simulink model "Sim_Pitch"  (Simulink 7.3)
settings: Solver=ode45  StartTime=0.0  StopTime=50  RelTol=1e-3
StartFcn:
  | [Avp, Bvp, Cvp, Dvp]= vehi_pdes;
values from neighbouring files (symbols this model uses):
  d2r = pi/180    (= 0.0174532925199)    [run.m]
  r2d = 180/pi    (= 57.2957795131)    [Pl.m]    (also in run.m)
undefined symbols (not defined in the file or in its folder): Avp, Bvp, Cvp, Dvp

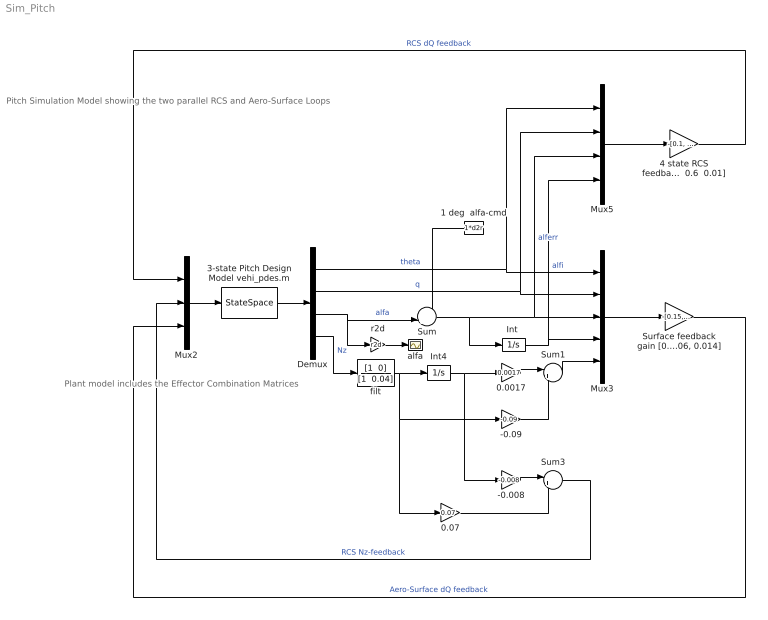
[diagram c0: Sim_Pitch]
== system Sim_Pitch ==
  note: Pitch Simulation Model showing the two parallel RCS and Aero-Surface Loops
  note: Plant model includes the Effector Combination Matrices
  -0.008 : Gain  Gain=-0.008  ParameterDataType=sfix(16)  ParameterScaling=2^0  OutDataType=sfix(16)  OutScaling=2^0
  -0.09 : Gain  Gain=-0.09  ParameterDataType=sfix(16)  ParameterScaling=2^0  OutDataType=sfix(16)  OutScaling=2^0
  0.0017 : Gain  Gain=0.0017  ParameterDataType=sfix(16)  ParameterScaling=2^0  OutDataType=sfix(16)  OutScaling=2^0
  0.07 : Gain  Gain=0.07  ParameterDataType=sfix(16)  ParameterScaling=2^0  OutDataType=sfix(16)  OutScaling=2^0
  1 deg  alfa-cmd : Constant  Value=1*d2r  OutDataType=sfix(16)  OutScaling=2^0
  3-state Pitch Design Model vehi_pdes.m : StateSpace  A=Avp  B=Bvp  C=Cvp  D=Dvp
  4 state RCS feedback [0.15  1.8  0.6  0.01] : Gain  Gain="-[0.1,   1.8,   0.9,    0.01]"  Multiplication=Matrix(K*u)  ParameterDataType=sfix(16)  ParameterScaling=2^0  OutDataType=sfix(16)  OutScaling=2^0
  Demux : Demux
  "Int " : Integrator
  Int4 : Integrator
  Mux2 : Mux  Inputs=3
  Mux3 : Mux  Inputs=5
  Mux5 : Mux
  Sum : Sum  Inputs=-+|  OutDataType=sfix(16)  OutScaling=2^0
  Sum1 : Sum  Inputs=|++  OutDataType=sfix(16)  OutScaling=2^0
  Sum3 : Sum  Inputs=|++  OutDataType=sfix(16)  OutScaling=2^0
  "Surface feedback gain [0.15, 2, 0.9, 0.06, 0.014]" : Gain  Gain="-[0.15,   2,   0.9,    0.06,   0.015]"  Multiplication=Matrix(K*u)  ParameterDataType=sfix(16)  ParameterScaling=2^0  OutDataType=sfix(16)  OutScaling=2^0
  alfa : Scope
  filt : TransferFcn  Numerator="[1  0]"  Denominator="[1  0.04]"
  r2d : Gain  Gain=r2d  ParameterDataType=sfix(16)  ParameterScaling=2^0  OutDataType=sfix(16)  OutScaling=2^0
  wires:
  3-state Pitch Design Model vehi_pdes.m/1 -> Demux/1
  Mux2/1 -> 3-state Pitch Design Model vehi_pdes.m/1
  Demux/1 -> Mux3/1, Mux5/1  "theta"
  Demux/2 -> Mux3/2, Mux5/2  "q"
  "Int "/1 -> Mux3/4, Mux5/4  "alfi"
  Demux/4 -> filt/1  "Nz"
  Demux/3 -> Sum/2, r2d/1  "alfa"
  Sum/1 -> "Int "/1, Mux3/3, Mux5/3  "alferr"
  1 deg  alfa-cmd/1 -> Sum/1
  filt/1 -> Int4/1, -0.09/1, 0.07/1
  0.0017/1 -> Sum1/1
  -0.09/1 -> Sum1/2
  Int4/1 -> 0.0017/1, -0.008/1
  r2d/1 -> alfa/1
  Sum1/1 -> Mux3/5
  Mux5/1 -> 4 state RCS feedback [0.15  1.8  0.6  0.01]/1
  0.07/1 -> Sum3/2
  -0.008/1 -> Sum3/1
  4 state RCS feedback [0.15  1.8  0.6  0.01]/1 -> Mux2/1  "RCS dQ feedback"
  Mux3/1 -> "Surface feedback gain [0.15, 2, 0.9, 0.06, 0.014]"/1
  Sum3/1 -> Mux2/2  "RCS Nz-feedback"
  "Surface feedback gain [0.15, 2, 0.9, 0.06, 0.014]"/1 -> Mux2/3  "Aero-Surface dQ feedback"
